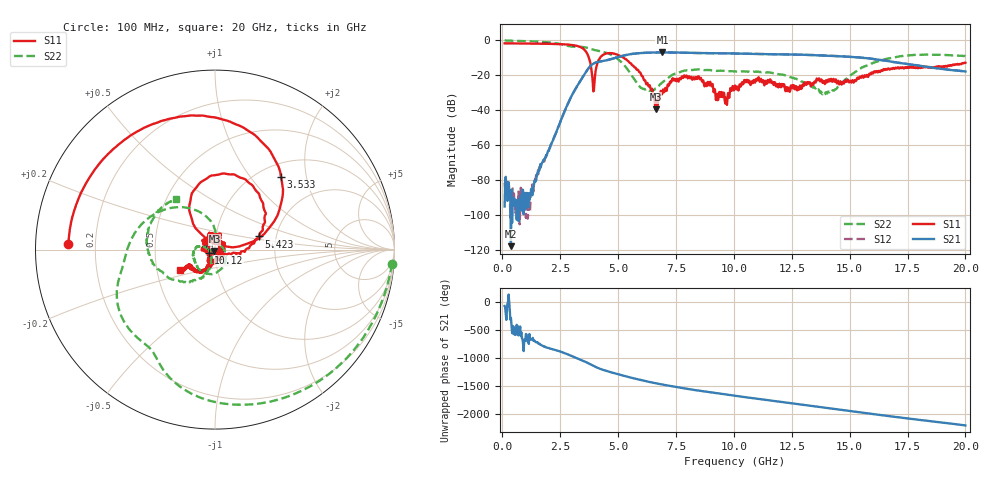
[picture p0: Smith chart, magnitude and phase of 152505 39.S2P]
!  2-Port S-parameters saved by WinCal
! VAR MeasName=S-Parameters (CALIBRATED_DATA) read from VNA (N5230C)
! VAR MeasDate=4/10/2015 9:32:21 AM
! VAR NAME=152505 39
! VAR FILENAME=152505 39.S2P
! VAR DATE=4/10/2015 9:32:21 AM
! VAR PHYS_PORTS=1,2
# Hz S DB R 50
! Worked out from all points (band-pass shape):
!   801 points, 100 MHz to 20 GHz, reference 50 ohm
!   highest |S21| = -6.94 dB at 6.916 GHz (marker M1); lowest = -118.0 dB at 373.6 MHz (marker M2)
!   |S21| within 3 dB of the highest: 4.907 GHz to 15.51 GHz (10.61 GHz wide, 104 % of centre)
!   lowest |S11| = -39.6 dB at 6.617 GHz (marker M3), VSWR 1.02, Z = 49.7 - j1.01 ohm
!   |S11| at or under -10 dB: 3.738 GHz to 4.219 GHz (481 MHz wide, 12.1 % of centre); 5.246 GHz to end of sweep
!   |S22| runs from -31.1 to -0.1 dB; largest |S21 - S12| = 0.0048
!   S11 on the Smith chart (normalised r, x): 100 MHz: 0.10, +0.02; 3.533 GHz: 1.25, +1.44; 5.423 GHz: 1.62, +0.25; 10.12 GHz: 0.93, -0.03; 20 GHz: 0.66, -0.16
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1e8  -1.75 177.7  -95.26 -66.7  -81.65 -133.5  -0.09 -4.5
3.73625e8  -1.77 171.1  -117.97 80.0  -90.60 -139.2  -0.21 -15.5
1.418375e9  -1.90 145.3  -80.78 20.8  -79.46 26.8  -0.68 -57.6
2.7865e9  -2.39 100.1  -37.67 155.1  -37.67 155.4  -3.09 -116.7
3.43325e9  -4.26 58.1  -21.90 43.1  -21.90 43.4  -3.77 -140.4
3.53275e9  -5.25 47.6  -19.76 25.6  -19.78 25.7  -3.92 -145.9
3.93075e9  -29.30 47.5  -13.41 -56.6  -13.41 -56.4  -5.38 -166.7
4.403375e9  -7.99 96.6  -11.70 -136.0  -11.73 -136.1  -6.79 168.7
5.42325e9  -11.85 16.7  -8.21 106.3  -8.20 106.3  -16.94 95.6
6.61725e9  -39.55 -105.8  -6.99 -7.7  -6.98 -7.8  -27.58 24.2
6.741625e9  -31.98 -161.0  -6.97 -17.9  -6.96 -18.1  -26.30 2.3
6.91575e9  -30.30 178.2  -6.94 -31.7  -6.96 -31.7  -24.05 -20.6
7.861e9  -20.08 109.1  -7.14 -100.3  -7.11 -100.1  -17.35 -92.5
8.70675e9  -25.00 72.2  -7.30 -154.4  -7.33 -154.6  -17.06 -127.2
9.70175e9  -37.01 -97.1  -7.49 147.2  -7.49 147.3  -17.68 -147.7
1.005e10  -25.89 -144.0  -7.54 127.1  -7.56 127.0  -17.85 -152.0
1.012462e10  -27.97 -152.4  -7.56 122.9  -7.59 123.1  -17.98 -153.5
1.19405e10  -26.43 64.5  -8.03 24.5  -8.05 24.6  -19.45 175.8
1.338325e10  -24.65 -77.6  -8.46 -53.1  -8.41 -52.9  -26.31 171.0
1.400512e10  -22.87 -109.5  -8.78 -86.9  -8.73 -86.9  -30.25 -154.8
1.669162e10  -16.22 -122.6  -11.97 124.2  -11.94 123.7  -10.38 -149.0
2e10  -12.86 -149.7  -17.85 -43.3  -17.80 -43.1  -9.05 127.5
